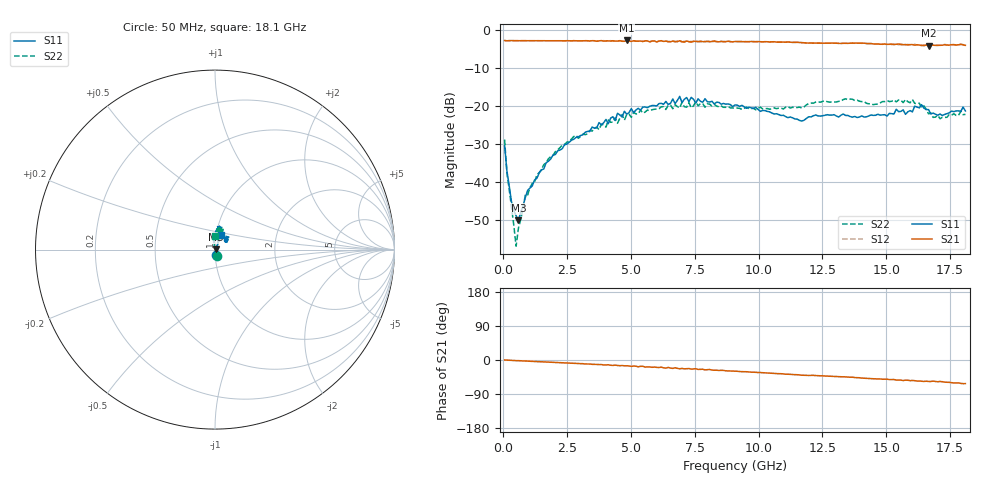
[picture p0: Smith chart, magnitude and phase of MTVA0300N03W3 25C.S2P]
! Network Analyzer HP8720D.06.14 Serial No. US36140669
!  7 Jul 2005  08:15:11
! Frequency  S11  S21  S12  S22
# HZ  S  DB R 50
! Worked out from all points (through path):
!   201 points, 50 MHz to 18.1 GHz, reference 50 ohm
!   highest |S21| = -2.79 dB at 4.833 GHz (marker M1); lowest = -4.2 dB at 16.66 GHz (marker M2)
!   group delay of S21, straight-line fit = 9.54 ps
!   lowest |S11| = -50.1 dB at 591.5 MHz (marker M3), VSWR 1.01, Z = 50.3 + j0.103 ohm
!   |S11| at or under -10 dB: start of sweep to end of sweep
!   |S22| runs from -56.8 to -18.1 dB; largest |S21 - S12| = 0.026
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5e7  -30.37 -74.8  -2.80 0.1  -2.83 0.1  -28.81 -67.8
1.4025e8  -37.08 -69.0  -2.88 -0.3  -2.87 -0.3  -37.66 -87.1
3.2075e8  -45.22 -50.2  -2.81 -0.8  -2.84 -0.8  -46.64 -97.9
5.0125e8  -48.84 -8.4  -2.86 -1.7  -2.84 -1.6  -56.82 -167.1
5.915e8  -50.06 19.1  -2.83 -1.7  -2.86 -1.8  -52.08 144.4
8.6225e8  -44.05 46.7  -2.85 -2.6  -2.86 -2.7  -43.26 130.5
1.58425e9  -36.53 60.4  -2.86 -5.0  -2.86 -5.1  -35.42 103.4
2.3965e9  -30.19 62.6  -2.88 -7.6  -2.87 -7.7  -30.10 97.3
3.1185e9  -27.56 68.1  -2.89 -9.7  -2.91 -10.0  -27.37 99.7
4.83325e9  -22.18 75.3  -2.79 -15.3  -2.90 -15.9  -22.24 83.9
6.09675e9  -19.37 73.5  -2.96 -19.8  -2.89 -19.7  -20.72 81.2
6.7285e9  -19.36 80.3  -3.05 -20.5  -3.21 -21.3  -19.64 74.5
6.909e9  -17.48 79.3  -2.86 -23.2  -2.97 -22.1  -20.50 73.6
7.54075e9  -19.22 75.5  -3.06 -23.1  -2.92 -24.9  -18.90 79.2
9.075e9  -19.72 85.6  -3.07 -29.5  -3.05 -29.5  -20.50 69.9
1.169225e10  -23.95 78.2  -3.37 -40.1  -3.37 -39.9  -20.54 79.5
1.21435e10  -22.57 73.9  -3.49 -40.5  -3.44 -40.6  -19.26 80.0
1.512175e10  -21.94 35.8  -3.80 -51.7  -3.67 -51.2  -18.84 81.4
1.602425e10  -21.55 46.8  -3.87 -54.0  -4.01 -55.8  -18.31 68.5
1.638525e10  -19.66 42.4  -4.15 -55.9  -3.96 -55.5  -20.44 64.8
1.6656e10  -20.95 43.4  -4.17 -56.6  -4.06 -55.7  -22.07 63.0
1.81e10  -21.30 65.9  -4.08 -62.2  -4.15 -63.2  -22.20 90.9
